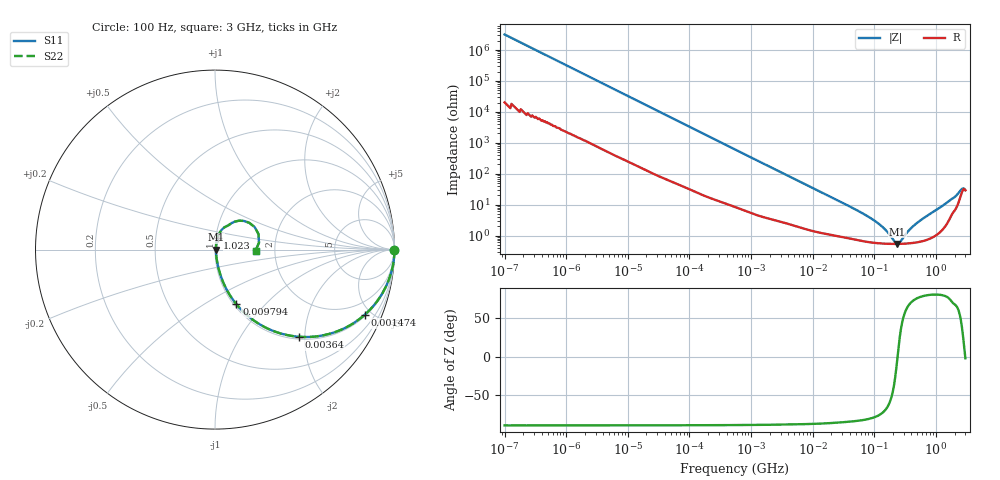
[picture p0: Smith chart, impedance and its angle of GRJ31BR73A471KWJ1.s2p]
!Murata Part Number: GRJ31BR73A471KWJ1
!These Parameters are Measured in Series Mode Connection
!Data Generated on Jun 19, 2026
!  o--ll--o
!Port1  Port2
!  o------o
!Operation Temp=25[degC], DC Bias Voltage=0[V]
!Freq. Start=100[Hz] Stop=3[GHz] 401[Steps]
# Hz S RI R 50
!Freq.(Hz) S11(Real) S11(Imag) S21(Real) S21(Imag) S12(Real) S12(Imag) S22(Real) S22(Imag)
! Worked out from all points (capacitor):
!   401 points, 100 Hz to 3 GHz, reference 50 ohm
!   read as one part in series: C = 498 pF near 109 Hz
!   lowest |Z| = 536 mohm at 236.7 MHz (marker M1)
!   series resonance near 237.7 MHz, so ESL is about 900 pH
!   S11 on the Smith chart (normalised r, x): 100 Hz: open; 1.474 MHz: 1.08, -4.56; 3.64 MHz: 1.05, -1.87; 9.794 MHz: 1.03, -0.70; 1.023 GHz: 1.02, +0.14; 3 GHz: 1.58, -0.02
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100  1 -3.13e-05  2e-07 3.13e-05  2e-07 3.13e-05  1 -3.13e-05
334  1 -0.000104  7e-07 0.000104  7e-07 0.000104  1 -0.000104
1788  1 -0.000553  4.3e-06 0.000553  4.3e-06 0.000553  1 -0.000553
31977  0.9998 -0.00975  0.000173 0.00975  0.000173 0.00975  0.9998 -0.00975
178874  0.9965 -0.0538  0.00346 0.0538  0.00346 0.0538  0.9965 -0.0538
547723  0.9717 -0.1592  0.0283 0.1592  0.0283 0.1592  0.9717 -0.1592
1473992  0.8343 -0.3629  0.1657 0.3629  0.1657 0.3629  0.8343 -0.3629
3639519  0.4663 -0.4855  0.5337 0.4855  0.5337 0.4855  0.4663 -0.4855
9794414  0.1196 -0.305  0.8804 0.305  0.8804 0.305  0.1196 -0.305
2.418395e7  0.0292 -0.1379  0.9708 0.1379  0.9708 0.1379  0.0292 -0.1379
7.405258e7  0.00816 -0.0435  0.9918 0.0435  0.9918 0.0435  0.00816 -0.0435
1.241234e8  0.00599 -0.0211  0.994 0.0211  0.994 0.0211  0.00599 -0.0211
1.751444e8  0.00544 -0.00944  0.9946 0.00944  0.9946 0.00944  0.00544 -0.00944
2.172002e8  0.00533 -0.00276  0.9947 0.00276  0.9947 0.00276  0.00533 -0.00276
2.36726e8  0.00533 -0.000124  0.9947 0.000124  0.9947 0.000124  0.00533 -0.000124
2.58007e8  0.00536 0.00251  0.9946 -0.00251  0.9946 -0.00251  0.00536 0.00251
4.514794e8  0.00627 0.0212  0.9937 -0.0212  0.9937 -0.0212  0.00627 0.0212
1.022825e9  0.0148 0.066  0.9852 -0.066  0.9852 -0.066  0.0148 0.066
1.642185e9  0.0464 0.1193  0.9536 -0.1193  0.9536 -0.1193  0.0464 0.1193
2.317205e9  0.1335 0.1609  0.8665 -0.1609  0.8665 -0.1609  0.1335 0.1609
2.636591e9  0.2211 0.1254  0.7789 -0.1254  0.7789 -0.1254  0.2211 0.1254
3e9  0.2258 -0.0062  0.7742 0.0062  0.7742 0.0062  0.2258 -0.0062
